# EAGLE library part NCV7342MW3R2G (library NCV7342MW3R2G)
Compatible with the ISO 11898-2, ISO 11898-5 Standards; High Speed (up to 1 Mbps); VIO Pin on NCV7342-3 Version Allowing Direct Interfacing with 3 V to 5 V Microcontrollers; VSPLIT Pin on NCV7342-0 Version for Bus Common Mode Stabilization; Very Low Current Consumption in Standby Mode with Wake-up via the Bus; Excellent EMS Level Over Full Frequency Range. Very Low EME. Low EME also without CM Choke.; Bus Pins Protected Against >15 kV System ESD Pulses; Transmit Data (TxD) Dominant Time-out Function; Bus Do Source: Datasheet
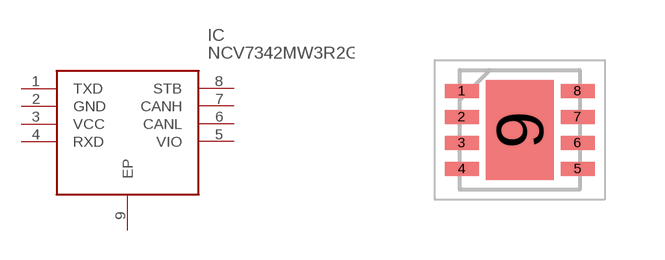
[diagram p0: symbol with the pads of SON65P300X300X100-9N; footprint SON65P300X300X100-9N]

Designator prefix IC

## NCV7342MW3R2G (Description: Compatible with the ISO 11898-2, ISO 11898-5 Standards; High Speed (up to 1 Mbps); VIO Pin on NCV7342-3 Version Allowing Direct Interfacing with 3 V to 5 V Microcontrollers; VSPLIT Pin on NCV7342-0 Version for Bus Common Mode Stabilization; Very Low Current Consumption in Standby Mode with Wake-up via the Bus; Excellent EMS Level Over Full Frequency Range. Very Low EME. Low EME also without CM Choke.; Bus Pins Protected Against >15 kV System ESD Pulses; Transmit Data (TxD) Dominant Time-out Function; Bus Do; Height: 1mm; Manufacturer_Name: onsemi; Manufacturer_Part_Number: NCV7342MW3R2G; Mouser_Part_Number: 863-NCV7342MW3R2G; Mouser_Price-Stock: https://www.mouser.co.uk/ProductDetail/onsemi/NCV7342MW3R2G?qs=z6PAvqrnkvRaXMr%2FitKpBw%3D%3D)  [SON65P300X300X100-9N]
1  TXD
2  GND
3  VCC
4  RXD
5  VIO
6  CANL
7  CANH
8  STB
9  EP

## Footprint SON65P300X300X100-9N (pad centres in mm)
DFN8, 3x3, 0.65P CASE 506DG ISSUE A
smd 0.85 x 0.35: 1 -1.45,0.975; 2 -1.45,0.325; 3 -1.45,-0.325; 4 -1.45,-0.975; 5 1.45,-0.975; 6 1.45,-0.325; 7 1.45,0.325; 8 1.45,0.975
smd 1.7 x 2.5: 9 0,0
